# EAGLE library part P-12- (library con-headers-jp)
HEADER PLUG PINS
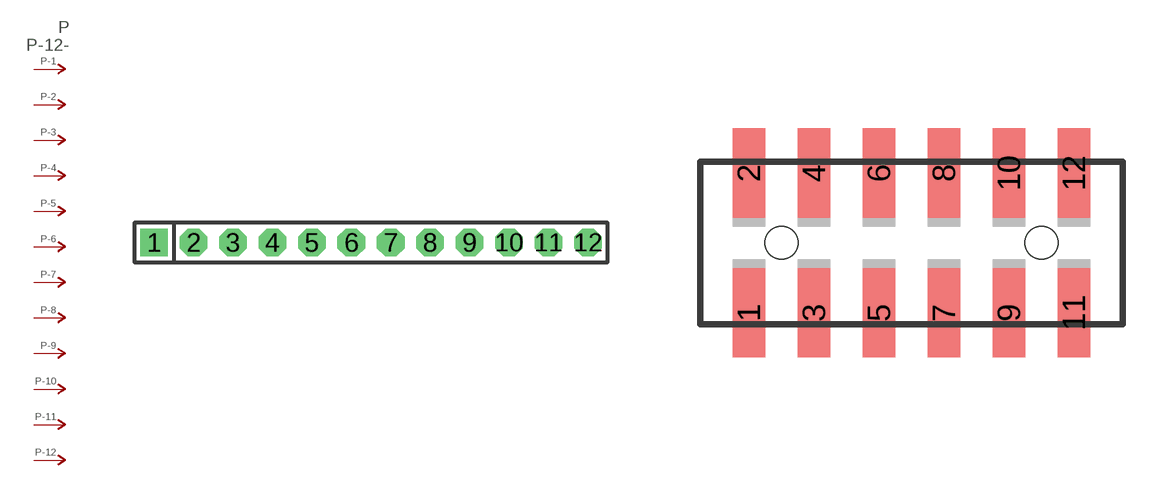
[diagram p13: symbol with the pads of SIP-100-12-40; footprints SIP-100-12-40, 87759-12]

Designator prefix P; gates -2=P-N -3=P-N -4=P-N -5=P-N -6=P-N -7=P-N -8=P-N -9=P-N -10=P-N -11=P-N -12=P-N -1=P-NV

## P-12-SIP-100-40  [SIP-100-12-40]
1  -1:P  pas
2  -2:P  pas
3  -3:P  pas
4  -4:P  pas
5  -5:P  pas
6  -6:P  pas
7  -7:P  pas
8  -8:P  pas
9  -9:P  pas
10  -10:P  pas
11  -11:P  pas
12  -12:P  pas

## P-12-87759  [87759-12]
Pads as for SIP-100-12-40

## P-12-100-2X06  [DIL-100-2X06]
Pads as for SIP-100-12-40

## P-12-100-2X06_M  [DIL-100-2X06_M]
Pads as for SIP-100-12-40

## P-12-2MM-2X06  [DIL-2MM-2X06]
Pads as for SIP-100-12-40

## P-12-2MM-2X06_M  [DIL-2MM-2X06_M]
Pads as for SIP-100-12-40

## P-12-SIP-100-32  [SIP-100-12-32]
Pads as for SIP-100-12-40

## P-12-SIP-100-40Y  [SIP-100-12-40Y]
Pads as for SIP-100-12-40

## P-12-SIP-100-32Y  [SIP-100-12-32Y]
Pads as for SIP-100-12-40

## P-12-87759_M  [87759-12_M]
Pads as for SIP-100-12-40

## P-12-LCW-112-XX-X-S  [LCW-112-XX-X-S]
Pads as for SIP-100-12-40

## P-12-LCW-112-XX-X-S-RE  [LCW-112-XX-X-S-RE]
Pads as for SIP-100-12-40

## Footprint SIP-100-12-40 (pad centres in mm)
SIP Header - 0.1", 40 mil drill
drill 1.016 pad 1.778 square: 1 -13.97,0
drill 1.016 pad 1.778 octagon: 2 -11.43,0; 3 -8.89,0; 4 -6.35,0; 5 -3.81,0; 6 -1.27,0; 7 1.27,0; 8 3.81,0; 9 6.35,0; 10 8.89,0; 11 11.43,0; 12 13.97,0

## Footprint 87759-12 (pad centres in mm)
Molex PCB Pin Headers 2.00mm (.079") Pitch Milli-Grid Header, Vertical SMD
smd 1 x 2.75: 1 -5,-2.15; 2 -5,2.15; 3 -3,-2.15; 4 -3,2.15; 5 -1,-2.15; 6 -1,2.15; 7 1,-2.15; 8 1,2.15; 9 3,-2.15; 10 3,2.15; 11 5,-2.15; 12 5,2.15
hole 1 at -4,0
hole 1 at 4,0

## Footprint DIL-100-2X06 (pad centres in mm)
PIN HEADER - 0.1"
drill 1.016 square: 1 -6.35,-1.27
drill 1.016 octagon: 2 -6.35,1.27; 3 -3.81,-1.27; 4 -3.81,1.27; 5 -1.27,-1.27; 6 -1.27,1.27; 7 1.27,-1.27; 8 1.27,1.27; 9 3.81,-1.27; 10 3.81,1.27; 11 6.35,-1.27; 12 6.35,1.27

## Footprint DIL-100-2X06_M (pad centres in mm)
PIN HEADER - MIRRORED 0.1"
drill 1.016 square: 1 -6.35,1.27
drill 1.016 octagon: 2 -6.35,-1.27; 3 -3.81,1.27; 4 -3.81,-1.27; 5 -1.27,1.27; 6 -1.27,-1.27; 7 1.27,1.27; 8 1.27,-1.27; 9 3.81,1.27; 10 3.81,-1.27; 11 6.35,1.27; 12 6.35,-1.27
